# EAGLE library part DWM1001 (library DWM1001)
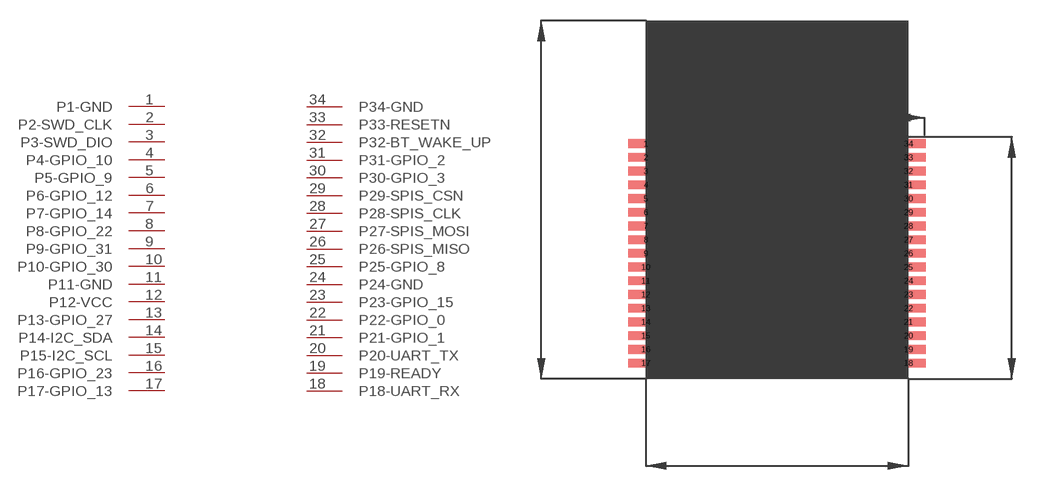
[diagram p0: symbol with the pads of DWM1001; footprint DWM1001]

Designator prefix -

## DWM1001  [DWM1001]
1  P1-GND  pwr
2  P2-SWD_CLK  in
3  P3-SWD_DIO
4  P4-GPIO_10
5  P5-GPIO_9
6  P6-GPIO_12
7  P7-GPIO_14
8  P8-GPIO_22
9  P9-GPIO_31
10  P10-GPIO_30
11  P11-GND  pwr
12  P12-VCC  pwr
13  P13-GPIO_27
14  P14-I2C_SDA
15  P15-I2C_SCL  out
16  P16-GPIO_23
17  P17-GPIO_13
18  P18-UART_RX  in
19  P19-READY  out
20  P20-UART_TX  out
21  P21-GPIO_1
22  P22-GPIO_0
23  P23-GPIO_15
24  P24-GND  pwr
25  P25-GPIO_8
26  P26-SPIS_MISO  in
27  P27-SPIS_MOSI  out
28  P28-SPIS_CLK  in
29  P29-SPIS_CSN  in
30  P30-GPIO_3
31  P31-GPIO_2
32  P32-BT_WAKE_UP  in
33  P33-RESETN  in
34  P34-GND  pwr

## Footprint DWM1001 (pad centres in mm)
smd 2.54 x 0.635: 1 0,17.15; 2 0,16.15; 3 0,15.15; 4 0,14.15; 5 0,13.15; 6 0,12.15; 7 0,11.15; 8 0,10.15; 9 0,9.15; 10 0,8.15; 11 0,7.15; 12 0,6.15; 13 0,5.15; 14 0,4.15; 15 0,3.15; 16 0,2.15; 17 0,1.15; 18 19.13,1.15; 19 19.13,2.15; 20 19.13,3.15; 21 19.13,4.15; 22 19.13,5.15; 23 19.13,6.15; 24 19.13,7.15; 25 19.13,8.15; 26 19.13,9.15; 27 19.13,10.15; 28 19.13,11.15; 29 19.13,12.15; 30 19.13,13.15; 31 19.13,14.15; 32 19.13,15.15; 33 19.13,16.15; 34 19.13,17.15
